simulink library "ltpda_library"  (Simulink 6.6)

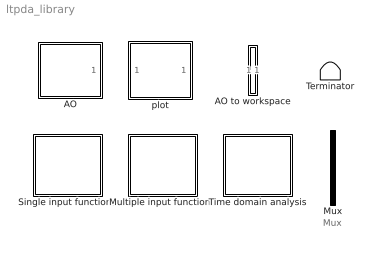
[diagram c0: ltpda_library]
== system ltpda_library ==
  note: Mux
  AO : Subsystem  Tag=input
  AO to workspace : Subsystem
  Multiple input functions : Subsystem
  Mux : Mux  Tag=mux  Inputs=2
  Single input functions : Subsystem
  Terminator : Terminator
  Time domain analysis : Subsystem
  plot : Subsystem

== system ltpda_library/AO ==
  Input : Constant
  Input AO : Outport
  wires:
  Input/1 -> Input AO/1

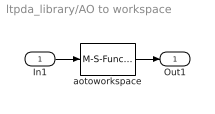
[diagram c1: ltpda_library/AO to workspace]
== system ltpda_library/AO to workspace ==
  In1 : Inport
  aotoworkspace : M-S-Function  Tag=ltpda_pwelch  FunctionName=aotoworkspace
  Out1 : Outport
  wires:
  aotoworkspace/1 -> Out1/1
  In1/1 -> aotoworkspace/1

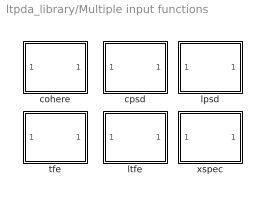
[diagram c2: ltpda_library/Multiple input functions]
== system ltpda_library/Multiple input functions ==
  cohere : Subsystem  Tag=function
  cpsd : Subsystem  Tag=function
  lpsd : Subsystem  Tag=function
  ltfe : Subsystem  Tag=function
  tfe : Subsystem  Tag=function
  xspec : Subsystem  Tag=function

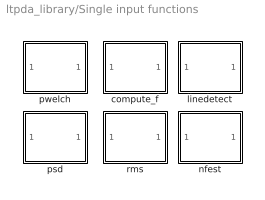
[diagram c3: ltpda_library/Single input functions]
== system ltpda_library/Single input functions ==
  compute_f : Subsystem  Tag=function
  linedetect : Subsystem  Tag=function
  nfest : Subsystem  Tag=function
  psd : Subsystem  Tag=function
  pwelch : Subsystem  Tag=function
  rms : Subsystem  Tag=function

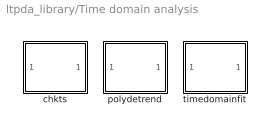
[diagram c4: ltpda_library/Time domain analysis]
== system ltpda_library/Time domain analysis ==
  chkts : Subsystem  Tag=function
  polydetrend : Subsystem  Tag=function
  timedomainfit : Subsystem  Tag=function

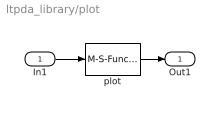
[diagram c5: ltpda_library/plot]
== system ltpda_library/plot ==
  In1 : Inport
  plot : M-S-Function  Tag=ltpda_tfe  FunctionName=ltpdaplot
  Out1 : Outport
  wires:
  In1/1 -> plot/1
  plot/1 -> Out1/1

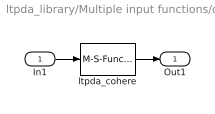
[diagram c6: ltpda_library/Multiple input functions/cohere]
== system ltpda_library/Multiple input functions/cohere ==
  In1 : Inport
  ltpda_cohere : M-S-Function  Tag=ltpda_cohere  FunctionName=ltpdasim
  Out1 : Outport
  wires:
  ltpda_cohere/1 -> Out1/1
  In1/1 -> ltpda_cohere/1

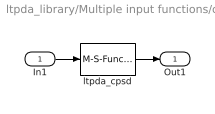
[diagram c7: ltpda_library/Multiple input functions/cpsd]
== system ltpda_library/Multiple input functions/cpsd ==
  In1 : Inport
  ltpda_cpsd : M-S-Function  Tag=ltpda_cpsd  FunctionName=ltpdasim
  Out1 : Outport
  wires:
  ltpda_cpsd/1 -> Out1/1
  In1/1 -> ltpda_cpsd/1

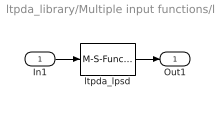
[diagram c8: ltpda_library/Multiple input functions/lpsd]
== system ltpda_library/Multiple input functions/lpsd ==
  In1 : Inport
  ltpda_lpsd : M-S-Function  Tag=ltpda_lpsd  FunctionName=ltpdasim
  Out1 : Outport
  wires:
  In1/1 -> ltpda_lpsd/1
  ltpda_lpsd/1 -> Out1/1

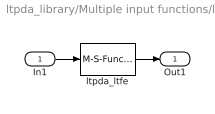
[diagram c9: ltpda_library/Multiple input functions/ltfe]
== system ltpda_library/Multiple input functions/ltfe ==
  In1 : Inport
  ltpda_ltfe : M-S-Function  Tag=ltpda_ltfe  FunctionName=ltpdasim
  Out1 : Outport
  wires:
  In1/1 -> ltpda_ltfe/1
  ltpda_ltfe/1 -> Out1/1

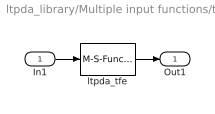
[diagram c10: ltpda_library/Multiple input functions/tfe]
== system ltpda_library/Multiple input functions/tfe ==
  In1 : Inport
  ltpda_tfe : M-S-Function  Tag=ltpda_tfe  FunctionName=ltpdasim
  Out1 : Outport
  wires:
  ltpda_tfe/1 -> Out1/1
  In1/1 -> ltpda_tfe/1

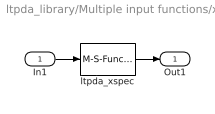
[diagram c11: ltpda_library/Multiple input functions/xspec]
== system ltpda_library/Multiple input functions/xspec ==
  In1 : Inport
  ltpda_xspec : M-S-Function  Tag=ltpda_xspec  FunctionName=ltpdasim
  Out1 : Outport
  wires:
  ltpda_xspec/1 -> Out1/1
  In1/1 -> ltpda_xspec/1

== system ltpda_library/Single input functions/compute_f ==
  In1 : Inport
  ltpda_compute_f : M-S-Function  Tag=ltpda_compute_f  FunctionName=ltpdasim
  Out1 : Outport
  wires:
  ltpda_compute_f/1 -> Out1/1
  In1/1 -> ltpda_compute_f/1

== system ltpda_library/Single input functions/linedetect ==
  In1 : Inport
  ltpda_linedetect : M-S-Function  Tag=ltpda_linedetect  FunctionName=ltpdasim
  Out1 : Outport
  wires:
  In1/1 -> ltpda_linedetect/1
  ltpda_linedetect/1 -> Out1/1

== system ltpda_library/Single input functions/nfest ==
  In1 : Inport
  ltpda_nfest : M-S-Function  Tag=ltpda_nfest  FunctionName=ltpdasim
  Out1 : Outport
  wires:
  ltpda_nfest/1 -> Out1/1
  In1/1 -> ltpda_nfest/1

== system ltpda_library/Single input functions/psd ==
  In1 : Inport
  ltpda_psd : M-S-Function  Tag=ltpda_psd  FunctionName=ltpdasim
  Out1 : Outport
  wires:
  ltpda_psd/1 -> Out1/1
  In1/1 -> ltpda_psd/1

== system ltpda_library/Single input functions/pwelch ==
  In1 : Inport
  ltpda_pwelch : M-S-Function  Tag=ltpda_pwelch  FunctionName=ltpdasim
  Out1 : Outport
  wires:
  In1/1 -> ltpda_pwelch/1
  ltpda_pwelch/1 -> Out1/1

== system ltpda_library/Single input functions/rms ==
  In1 : Inport
  ltpda_rms : M-S-Function  Tag=ltpda_rms  FunctionName=ltpdasim
  Out1 : Outport
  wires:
  In1/1 -> ltpda_rms/1
  ltpda_rms/1 -> Out1/1

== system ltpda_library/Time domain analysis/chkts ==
  In1 : Inport
  ltpda_chkts : M-S-Function  Tag=ltpda_chkts  FunctionName=ltpdasim
  Out1 : Outport
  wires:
  ltpda_chkts/1 -> Out1/1
  In1/1 -> ltpda_chkts/1

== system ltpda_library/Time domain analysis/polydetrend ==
  In1 : Inport
  ltpda_polydetrend : M-S-Function  Tag=ltpda_polydetrend  FunctionName=ltpdasim
  Out1 : Outport
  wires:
  In1/1 -> ltpda_polydetrend/1
  ltpda_polydetrend/1 -> Out1/1

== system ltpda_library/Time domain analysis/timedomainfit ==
  In1 : Inport
  ltpda_timedomainfit : M-S-Function  Tag=ltpda_timedomainfit  FunctionName=ltpdasim
  Out1 : Outport
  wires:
  ltpda_timedomainfit/1 -> Out1/1
  In1/1 -> ltpda_timedomainfit/1
